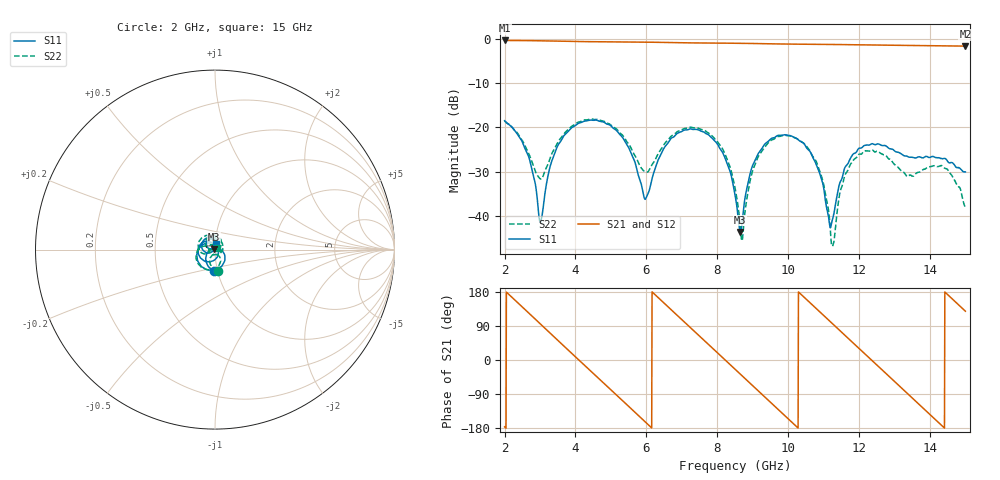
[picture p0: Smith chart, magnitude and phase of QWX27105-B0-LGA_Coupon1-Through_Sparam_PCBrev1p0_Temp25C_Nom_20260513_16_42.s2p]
! S2P file generated by MATLAB
! VNA used: R&S ZNB40
! calKit used: Agilent 85052D 3.5mm Calibration Kit
! Date of calibration: 2026 05 13,  4:42 PM
! Date of measurement: 2026 05 13,  4:42 PM
! Data order: f(GHz) S11(dB,degree) S21(dB,degree) S12(dB,degree) S22(dB,degree)
# GHz S DB R 50.00
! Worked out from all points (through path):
!   1301 points, 2 GHz to 15 GHz, reference 50 ohm
!   highest |S21| = -0.40 dB at 2 GHz (marker M1); lowest = -1.7 dB at 15 GHz (marker M2)
!   group delay of S21, straight-line fit = 242 ps
!   lowest |S11| = -43.7 dB at 8.65 GHz (marker M3), VSWR 1.01, Z = 49.4 + j0.185 ohm
!   |S11| at or under -10 dB: start of sweep to end of sweep
!   |S22| runs from -46.8 to -18.1 dB; largest |S21 - S12| = 0.008
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2  -18.52 -93.7  -0.40 -176.4  -0.42 -176.4  -18.58 -82.9
2.66  -26.22 -156.0  -0.44 125.8  -0.45 125.8  -25.59 -120.2
3.02  -41.34 89.9  -0.48 94.1  -0.48 94.2  -31.69 -86.0
3.45  -25.03 -24.5  -0.53 56.4  -0.53 56.4  -24.19 -61.0
4.17  -18.88 -92.2  -0.65 -6.6  -0.65 -6.5  -18.61 -106.8
5.2  -21.13 173.7  -0.73 -96.1  -0.74 -96.2  -20.77 178.4
5.97  -36.26 29.2  -0.78 -163.5  -0.79 -163.6  -30.02 -177.5
6.34  -27.23 -73.0  -0.82 164.0  -0.83 164.0  -25.80 -153.3
7.32  -20.50 -170.2  -0.95 78.7  -0.97 78.6  -20.12 147.7
7.95  -23.29 136.5  -1.00 23.9  -1.02 23.7  -22.80 97.7
8.5  -35.23 108.0  -1.03 -24.3  -1.05 -24.3  -33.63 60.5
8.65  -43.66 163.4  -1.05 -37.5  -1.06 -37.4  -42.89 86.7
8.98  -28.98 -148.3  -1.08 -66.1  -1.10 -66.5  -30.29 177.3
9.5  -22.68 174.0  -1.16 -111.7  -1.17 -111.7  -23.04 138.9
10.11  -22.06 126.3  -1.23 -164.8  -1.24 -164.8  -22.07 89.3
10.67  -26.33 85.7  -1.26 146.4  -1.28 146.5  -26.23 42.3
11.26  -40.57 159.1  -1.31 95.0  -1.32 94.9  -46.67 97.1
11.79  -26.56 160.7  -1.37 48.7  -1.38 48.5  -28.02 111.1
12.84  -24.75 103.3  -1.48 -42.6  -1.49 -43.0  -27.17 6.1
13.46  -26.75 93.3  -1.53 -96.7  -1.54 -97.1  -30.81 -104.0
14.12  -26.72 85.8  -1.59 -154.4  -1.60 -154.7  -28.69 150.6
15  -30.07 77.0  -1.68 128.8  -1.68 128.7  -38.23 30.3
